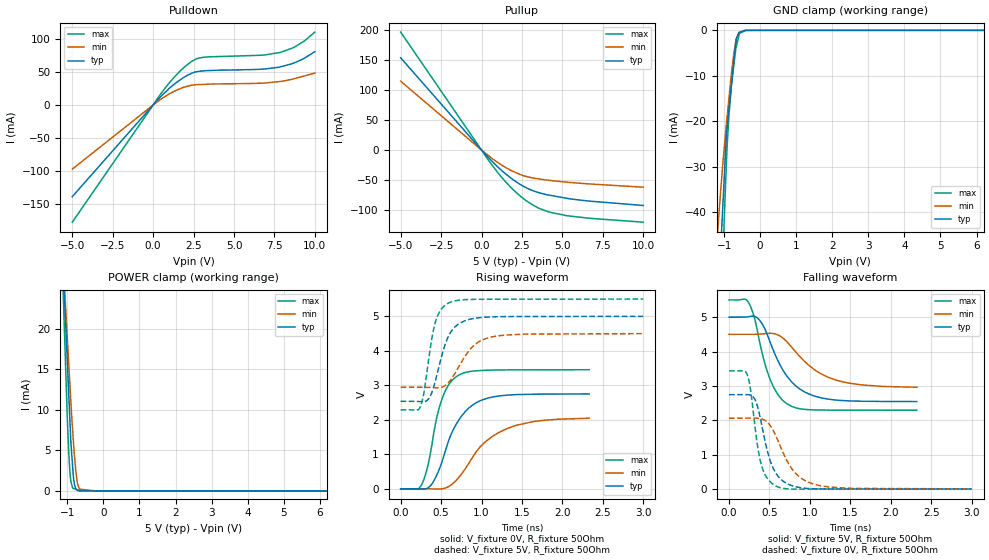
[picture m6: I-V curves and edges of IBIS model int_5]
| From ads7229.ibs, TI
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|   int_5 Model
[Model]   int_5
Model_type   I/O
Polarity   Non-Inverting
Enable   Active-Low
Vinl = 1.75
Vinh = 3.25
Vmeas = 2.5
Vref = 2.5
Cref = 30pF
Rref = 50
|   typ   min   max
|   (nom PVT)   (Fast PVT)   (slow PVT)
|C_comp from frequency sweep method(F=50MHz)
C_comp   4.855e-12   3.896e-12   5.693e-12
|OFF state: BUFFER IN HIGH IMPEDANCE
|C_comp   4.855e-12   3.896e-12   5.693e-12
|ON state : BUFFER OUTPUT TURNED HIGH
|C_comp   5.192e-12   4.233e-12   6.095e-12
|C_comp from LC tank measurement(L=1nH)
|ON state : BUFFER OUTPUT TURNED HIGH
|Resonant Frequency(Hz)   2.480e+09   2.680e+09   2.370e+09
|C_comp   4.123e-12   3.530e-12   4.514e-12
|OFF state: BUFFER IN HIGH IMPEDANCE
|Resonant Frequency   2.600e+09   2.850e+09   2.440e+09
|C_comp   3.751e-12   3.122e-12   4.259e-12
| Where nom  PVT is Nominal Process,  5V,  28C
|   Fast PVT is Strong Process,   5.5V,  -40C
|   Slow PVT is Weak Process,   4.5V,  88C
[Model Spec]
|Subparameter   typ   min   max
Vinh   3.25   2.925   3.575
Vinl   1.75   1.575   1.925
[Voltage Range]   5   4.5   5.5
|Ambient Temperature   25   85   -40
|Junction Temperature
[Temperature Range]   28   88   -40
[Pullup Reference]   5   4.5   5.5
[Pulldown Reference]   0   0   0
[Power Clamp Reference]   5   4.5   5.5
[GND Clamp Reference]   0   0   0
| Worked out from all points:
|   slope of the pulldown table from 0 to 0.75 V, typ, clamps not added: 38.9 ohm
|   slope of the pullup table from 0 to 0.75 V, typ, clamps not added: 35.2 ohm
|   GND clamp passes 1 mA (typ) near -0.62 V on its own axis
|   POWER clamp passes 1 mA (typ) near -0.81 V on its own axis
|   falling waveform, V_fixture 5V, R_fixture 50Ohm: 20-80 % time 340ps typ, 460ps min, 231ps max; typ from 5 V to 2.55 V
|   rising waveform, V_fixture 0V, R_fixture 50Ohm: 20-80 % time 311ps typ, 473ps min, 199ps max; typ from 0 V to 2.75 V
|   rising waveform, V_fixture 5V, R_fixture 50Ohm: 20-80 % time 193ps typ, 276ps min, 135ps max; typ from 2.53 V to 5 V
|   falling waveform, V_fixture 0V, R_fixture 50Ohm: 20-80 % time 184ps typ, 283ps min, 129ps max; typ from 2.75 V to 0.009 V
[Pulldown]
|   Voltage   I(typ)   I(min)   I(max)
-5V       -138.4mA   -96.83mA   -177mA
528mV     14.11mA    9.495mA    18.76mA
1.216V    29.73mA    19.67mA    39.74mA
2.007V    43.3mA     27.58mA    58.86mA
2.38V     47.96mA    29.92mA    65.81mA
2.684V    50.17mA    30.7mA     69.91mA
3.08V     51.49mA    31.09mA    71.99mA
6.6V      53.94mA    32.88mA    75.06mA
7.854V    57.55mA    35.54mA    79.3mA
8.684V    63.33mA    39.47mA    86.72mA
9.35V     70.62mA    43.89mA    96.59mA
10V       80.52mA    48.22mA    110.1mA
[GND Clamp]
|   Voltage   I(typ)   I(min)   I(max)
-5V       -892.6mA   -646.6mA   -1.244A
-1.216V   -69.01mA   -48.87mA   -99.62mA
-1.143V   -55.86mA   -40.33mA   -79.34mA
-1.089V   -47.18mA   -34.62mA   -64.72mA
-1.044V   -40mA      -30.13mA   -53.41mA
-1.001V   -33.15mA   -26.25mA   -42.6mA
-935mV    -22.86mA   -20.46mA   -28.8mA
-863.5mV  -17.25mA   -14.75mA   -18.41mA
-786.5mV  -11.21mA   -8.852mA   -11.26mA
-670mV    -2.069mA   -2.242mA   -3.888mA
-580.5mV  -549.3uA   -384.9uA   -836.4uA
10V       0A         0A         0A
[Pullup]
|   Voltage   I(typ)   I(min)   I(max)
-5V       153.8mA    114.8mA    196.7mA
445.5mV   -13.17mA   -9.806mA   -17.57mA
1.04V     -28.95mA   -21.46mA   -38.79mA
1.672V    -43.61mA   -31.8mA    -58.38mA
2.475V    -58.65mA   -41.69mA   -78.57mA
3.08V     -66.79mA   -46.16mA   -90.21mA
3.52V     -70.95mA   -48.04mA   -96.68mA
4.301V    -75.82mA   -50.92mA   -104.2mA
5.192V    -80.1mA    -53.4mA    -109.1mA
6.6V      -84.95mA   -56.4mA    -113.6mA
10V       -92.49mA   -61.96mA   -120.4mA
[POWER Clamp]
|   Voltage   I(typ)   I(min)   I(max)
-5V       207.8mA    188.7mA    235.2mA
-1.14V    29.98mA    30.25mA    28.15mA
-1.111V   27.05mA    27.69mA    23.81mA
-1.098V   25.73mA    26.55mA    22.03mA
-1.001V   15.92mA    18.78mA    8.86mA
-929.5mV  8.681mA    13.06mA    2.319mA
-900mV    5.812mA    10.7mA     1.118mA
-835mV    1.822mA    6.276mA    318.4uA
-720mV    59.67uA    941.3uA    122.5uA
-666mV    12.26uA    216.5uA    30.46uA
-202.5mV  0A         0A         466.9nA
10V       0A         0A         0A
[Ramp]
R_load = 50
|   typ   min   max
dV/dt_r   1.65043/3.10328e-10   1.23462/4.79536e-10   2.07117/1.98522e-10
dV/dt_f   1.47293/3.39241e-10   0.92763/4.63331e-10   1.92412/2.31099e-10
[Falling Waveform]
V_fixture = 5V
V_fixture_min = 4.5V
V_fixture_max = 5.5V
R_fixture = 50Ohm
|   Time   V(typ)   V(min)   V(max)
0s        5V         4.5V       5.5V
244ps     5.011V     4.499V     5.414V
306ps     5.025V     4.5V       5.049V
372ps     4.928V     4.506V     4.35V
511ps     4.257V     4.532V     3.176V
601ps     3.752V     4.485V     2.764V
714ps     3.291V     4.291V     2.487V
942ps     2.819V     3.695V     2.319V
1.317ns   2.592V     3.176V     2.299V
2.322ns   2.548V     2.963V     2.295V
[Rising Waveform]
V_fixture = 0V
V_fixture_min = 0V
V_fixture_max = 0V
R_fixture = 50Ohm
|   Time   V(typ)   V(min)   V(max)
0s        1.65nV     1.848nV    1.527nV
262ps     -6.345mV   634uV      130mV
340ps     30.82mV    -362.2uV   700.2mV
439ps     358.2mV    -5.785mV   1.985V
490ps     641mV      -3.841mV   2.449V
582ps     1.312V     50.75mV    2.971V
689ps     1.878V     250.4mV    3.25V
938ps     2.497V     1.084V     3.419V
1.326ns   2.716V     1.755V     3.445V
2.331ns   2.749V     2.045V     3.45V
[Rising Waveform]
V_fixture = 5V
V_fixture_min = 4.5V
V_fixture_max = 5.5V
R_fixture = 50Ohm
|   Time   V(typ)   V(min)   V(max)
0s        2.534V     2.941V     2.288V
246ps     2.525V     2.942V     2.39V
287ps     2.521V     2.941V     2.778V
344ps     2.602V     2.938V     3.708V
427ps     3.104V     2.93V      4.811V
497ps     3.753V     2.938V     5.185V
602ps     4.469V     3.104V     5.393V
875ps     4.923V     4.084V     5.487V
1.129ns   4.981V     4.401V     5.492V
3ns       4.996V     4.495V     5.497V
[Falling Waveform]
V_fixture = 0V
V_fixture_min = 0V
V_fixture_max = 0V
R_fixture = 50Ohm
|   Time   V(typ)   V(min)   V(max)
0s        2.748V     2.065V     3.44V
222ps     2.749V     2.066V     3.352V
267ps     2.733V     2.067V     2.87V
324ps     2.594V     2.067V     1.768V
394ps     1.988V     2.049V     760.7mV
499ps     899mV      1.881V     244mV
586ps     442mV      1.513V     87.24mV
806ps     84.4mV     508.7mV    3.608mV
1.056ns   12.97mV    142.9mV    7.876mV
3ns       8.925mV    11.47mV    5.009mV
